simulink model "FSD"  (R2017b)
settings: Solver=FixedStepDiscrete  StartTime=0.0  StopTime=10.0  FixedStep=0.01  RelTol=1e-3  EnableMultiTasking=on
undefined symbols (not defined in the file): ASWTYPE_FALSE, ASWTYPE_TRUE, CcFSD_MSDOpenFltDelTi_ms, CcFSD_MSDOpenPackVolt_V, CcFSD_MSDOpenSumCellVolt_V, FSD_RUNTIME_MS
libraries: AIWAYS_Powertrain_BMS_lib x6

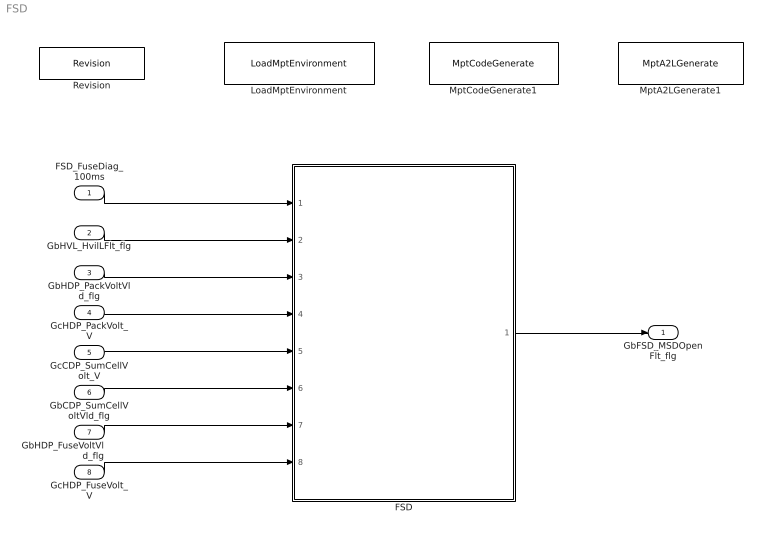
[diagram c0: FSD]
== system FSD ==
  FSD_FuseDiag_100ms : Inport
  GbHVL_HvilLFlt_flg : Inport  Port=2
  GbHDP_PackVoltVld_flg : Inport  Port=3
  GcHDP_PackVolt_V : Inport  Port=4
  GcCDP_SumCellVolt_V : Inport  Port=5
  GbCDP_SumCellVoltVld_flg : Inport  Port=6
  GbHDP_FuseVoltVld_flg : Inport  Port=7
  GcHDP_FuseVolt_V : Inport  Port=8
  FSD : Subsystem
  LoadMptEnvironment : AIWAYS_Powertrain_BMS_lib/Config/LoadMptEnvironment  ProjectName=Comm  SuppierID=NewPlatformUAES
  MptA2LGenerate1 : AIWAYS_Powertrain_BMS_lib/Config/MptA2LGenerate  SystemSampleTime=-1
  MptCodeGenerate1 : AIWAYS_Powertrain_BMS_lib/Config/MptCodeGenerate  SystemSampleTime=-1
  Revision : AIWAYS_Powertrain_BMS_lib/Config/Revision  curVersion='M102C102R103'  newVersion='M102C102R103'
  GbFSD_MSDOpenFlt_flg : Outport
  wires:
  FSD_FuseDiag_100ms/1 -> FSD/1(FSD_FuseDiag_100ms)
  GbHVL_HvilLFlt_flg/1 -> FSD/2(GbHVL_HvilLFlt_flg)
  GbHDP_PackVoltVld_flg/1 -> FSD/3(GbHDP_PackVoltVld_flg)
  GcHDP_PackVolt_V/1 -> FSD/4(GcHDP_PackVolt_V)
  GcCDP_SumCellVolt_V/1 -> FSD/5(GcCDP_SumCellVolt_V)
  GbCDP_SumCellVoltVld_flg/1 -> FSD/6(GbCDP_SumCellVoltVld_flg)
  FSD/1(GbFSD_MSDOpenFlt_flg) -> GbFSD_MSDOpenFlt_flg/1
  GbHDP_FuseVoltVld_flg/1 -> FSD/7(GbHDP_FuseVoltVld_flg)
  GcHDP_FuseVolt_V/1 -> FSD/8(GcHDP_FuseVolt_V)

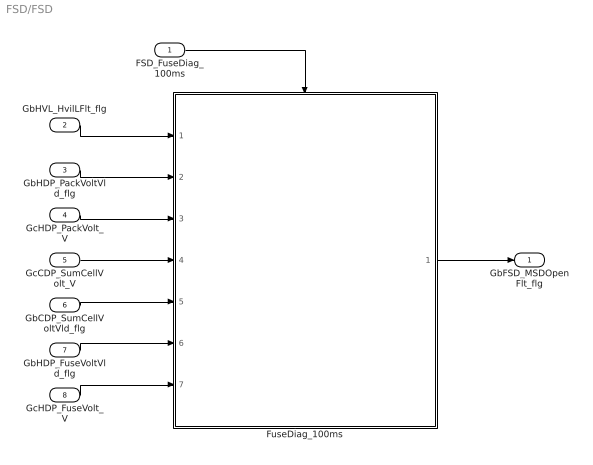
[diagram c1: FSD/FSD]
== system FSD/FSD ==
  FSD_FuseDiag_100ms : Inport
  GbHVL_HvilLFlt_flg : Inport  Port=2
  GbHDP_PackVoltVld_flg : Inport  Port=3
  GcHDP_PackVolt_V : Inport  Port=4
  GcCDP_SumCellVolt_V : Inport  Port=5
  GbCDP_SumCellVoltVld_flg : Inport  Port=6
  GbHDP_FuseVoltVld_flg : Inport  Port=7
  GcHDP_FuseVolt_V : Inport  Port=8
  FuseDiag_100ms : Subsystem
  GbFSD_MSDOpenFlt_flg : Outport
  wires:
  FSD_FuseDiag_100ms/1 -> FuseDiag_100ms/Trigger
  GbHDP_PackVoltVld_flg/1 -> FuseDiag_100ms/2(GbHDP_PackVoltVld_flg)
  GcHDP_PackVolt_V/1 -> FuseDiag_100ms/3(GcHDP_PackVolt_V)
  GbHVL_HvilLFlt_flg/1 -> FuseDiag_100ms/1(GbHVL_HvilLFlt_flg)
  GcCDP_SumCellVolt_V/1 -> FuseDiag_100ms/4(GcCDP_SumCellVolt_V)
  GbCDP_SumCellVoltVld_flg/1 -> FuseDiag_100ms/5(GbCDP_SumCellVoltVld_flg)
  FuseDiag_100ms/1(GbFSD_MSDOpenFlt_flg) -> GbFSD_MSDOpenFlt_flg/1
  GbHDP_FuseVoltVld_flg/1 -> FuseDiag_100ms/6(GbHDP_FuseVoltVld_flg)
  GcHDP_FuseVolt_V/1 -> FuseDiag_100ms/7(GcHDP_FuseVolt_V)

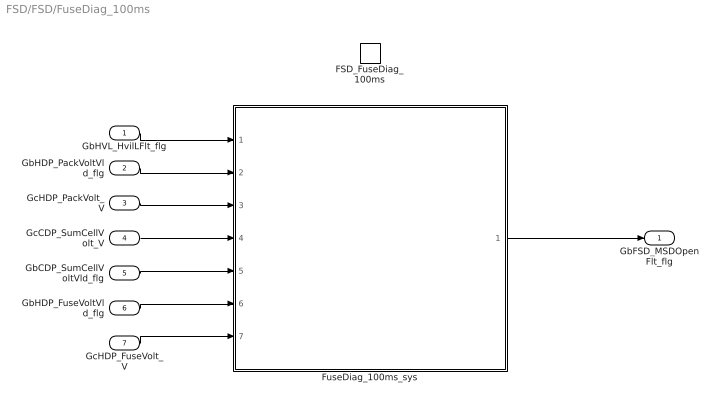
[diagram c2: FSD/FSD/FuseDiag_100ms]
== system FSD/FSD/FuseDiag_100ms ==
  GbHVL_HvilLFlt_flg : Inport
  GbHDP_PackVoltVld_flg : Inport  Port=2
  GcHDP_PackVolt_V : Inport  Port=3
  GcCDP_SumCellVolt_V : Inport  Port=4
  GbCDP_SumCellVoltVld_flg : Inport  Port=5
  GbHDP_FuseVoltVld_flg : Inport  Port=6
  GcHDP_FuseVolt_V : Inport  Port=7
  FSD_FuseDiag_100ms : TriggerPort  TriggerType=function-call  VariantControl=(inherit)
  FuseDiag_100ms_sys : Subsystem
  GbFSD_MSDOpenFlt_flg : Outport
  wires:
  GbHVL_HvilLFlt_flg/1 -> FuseDiag_100ms_sys/1(GbHVL_HvilLFlt_flg)
  GbHDP_PackVoltVld_flg/1 -> FuseDiag_100ms_sys/2(GbHDP_PackVoltVld_flg)
  GcHDP_PackVolt_V/1 -> FuseDiag_100ms_sys/3(GcHDP_PackVolt_V)
  GcCDP_SumCellVolt_V/1 -> FuseDiag_100ms_sys/4(GcCDP_SumCellVolt_V)
  GbCDP_SumCellVoltVld_flg/1 -> FuseDiag_100ms_sys/5(GbCDP_SumCellVoltVld_flg)
  FuseDiag_100ms_sys/1(GbFSD_MSDOpenFlt_flg) -> GbFSD_MSDOpenFlt_flg/1
  GbHDP_FuseVoltVld_flg/1 -> FuseDiag_100ms_sys/6(GbHDP_FuseVoltVld_flg)
  GcHDP_FuseVolt_V/1 -> FuseDiag_100ms_sys/7(GcHDP_FuseVolt_V)

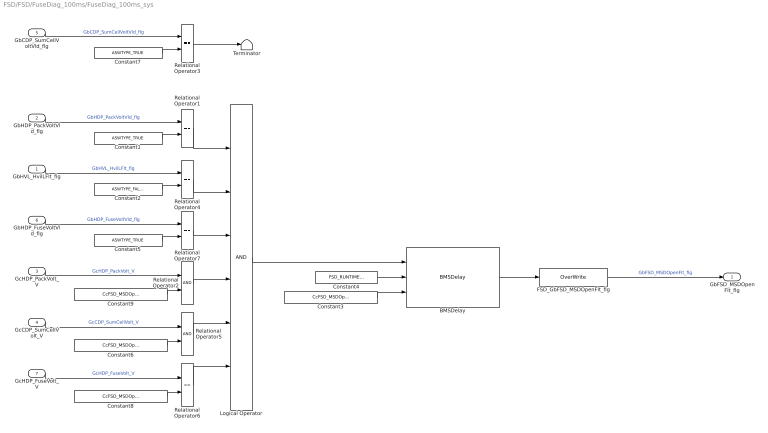
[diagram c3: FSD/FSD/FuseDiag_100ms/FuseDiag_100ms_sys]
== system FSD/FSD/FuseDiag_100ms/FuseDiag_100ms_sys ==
  GbHVL_HvilLFlt_flg : Inport
  GbHDP_PackVoltVld_flg : Inport  Port=2
  GcHDP_PackVolt_V : Inport  Port=3
  GcCDP_SumCellVolt_V : Inport  Port=4
  GbCDP_SumCellVoltVld_flg : Inport  Port=5
  GbHDP_FuseVoltVld_flg : Inport  Port=6
  GcHDP_FuseVolt_V : Inport  Port=7
  BMSDelay : AIWAYS_Powertrain_BMS_lib/Debounce & Delay/BMSDelay
  Constant1 : Constant  Value=ASWTYPE_TRUE
  Constant2 : Constant  Value=ASWTYPE_FALSE
  Constant3 : Constant  Value=CcFSD_MSDOpenFltDelTi_ms
  Constant4 : Constant  Value=FSD_RUNTIME_MS
  Constant5 : Constant  Value=ASWTYPE_TRUE
  Constant6 : Constant  Value=CcFSD_MSDOpenSumCellVolt_V
  Constant7 : Constant  Value=ASWTYPE_TRUE
  Constant8 : Constant  Value=CcFSD_MSDOpenPackVolt_V
  Constant9 : Constant  Value=CcFSD_MSDOpenSumCellVolt_V
  FSD_GbFSD_MSDOpenFlt_flg : AIWAYS_Powertrain_BMS_lib/Signals/OverWrite  OverWrite_Value=CbFSD_MSDOpenFltOvr_flg  OverWrite_flag=CbFSD_MSDOpenFltOvrSwt_flg
  Logical Operator : Logic  Inputs=6  AllPortsSameDT=off  OutDataTypeStr=boolean
  Relational Operator{1,3..4,7} (4 alike) : RelationalOperator  Operator===  OutDataTypeStr=boolean
  Relational Operator2 : RelationalOperator  OutDataTypeStr=boolean
  Relational Operator5 : RelationalOperator  OutDataTypeStr=boolean
  Relational Operator6 : RelationalOperator  Operator=<=  OutDataTypeStr=boolean
  Terminator : Terminator
  GbFSD_MSDOpenFlt_flg : Outport
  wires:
  Constant1/1 -> Relational Operator1/2
  GbHDP_PackVoltVld_flg/1 -> Relational Operator1/1  "GbHDP_PackVoltVld_flg"
  Constant7/1 -> Relational Operator3/2
  GbCDP_SumCellVoltVld_flg/1 -> Relational Operator3/1  "GbCDP_SumCellVoltVld_flg"
  Constant2/1 -> Relational Operator4/2
  GbHVL_HvilLFlt_flg/1 -> Relational Operator4/1  "GbHVL_HvilLFlt_flg"
  GcHDP_PackVolt_V/1 -> Relational Operator2/1  "GcHDP_PackVolt_V"
  GcCDP_SumCellVolt_V/1 -> Relational Operator5/1  "GcCDP_SumCellVolt_V"
  Constant3/1 -> BMSDelay/3
  Logical Operator/1 -> BMSDelay/1
  Constant4/1 -> BMSDelay/2
  Relational Operator1/1 -> Logical Operator/1
  Relational Operator3/1 -> Terminator/1
  BMSDelay/1 -> FSD_GbFSD_MSDOpenFlt_flg/1
  Constant9/1 -> Relational Operator2/2
  Constant6/1 -> Relational Operator5/2
  FSD_GbFSD_MSDOpenFlt_flg/1 -> GbFSD_MSDOpenFlt_flg/1  "GbFSD_MSDOpenFlt_flg"
  Constant8/1 -> Relational Operator6/2
  Constant5/1 -> Relational Operator7/2
  GbHDP_FuseVoltVld_flg/1 -> Relational Operator7/1  "GbHDP_FuseVoltVld_flg"
  GcHDP_FuseVolt_V/1 -> Relational Operator6/1  "GcHDP_FuseVolt_V"
  Relational Operator4/1 -> Logical Operator/2
  Relational Operator7/1 -> Logical Operator/3
  Relational Operator2/1 -> Logical Operator/4
  Relational Operator5/1 -> Logical Operator/5
  Relational Operator6/1 -> Logical Operator/6
